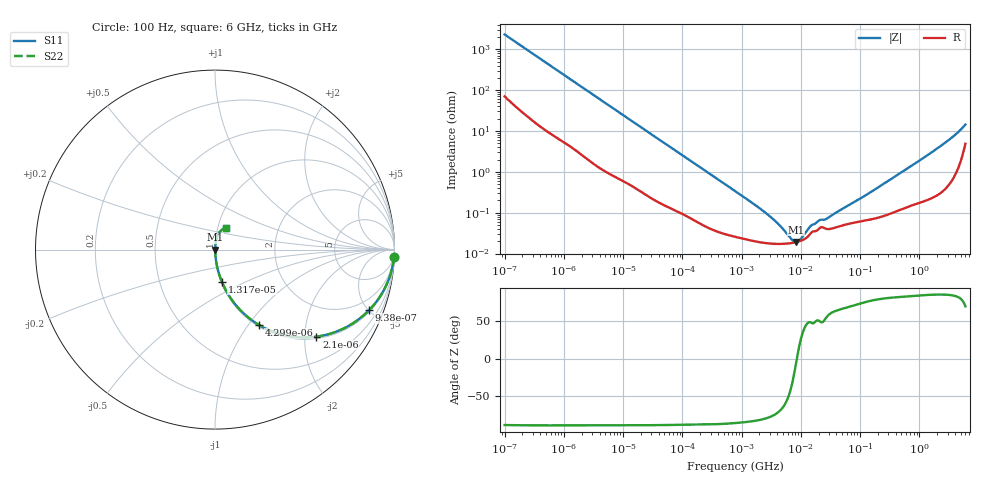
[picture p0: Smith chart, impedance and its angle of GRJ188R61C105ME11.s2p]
!Murata Part Number: GRJ188R61C105ME11
!These Parameters are Measured in Series Mode Connection
!Data Generated on Jun 19, 2026
!  o--ll--o
!Port1  Port2
!  o------o
!Operation Temp=25[degC], DC Bias Voltage=0[V]
!Freq. Start=100[Hz] Stop=6[GHz] 401[Steps]
# Hz S RI R 50
!Freq.(Hz) S11(Real) S11(Imag) S21(Real) S21(Imag) S12(Real) S12(Imag) S22(Real) S22(Imag)
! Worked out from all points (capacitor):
!   401 points, 100 Hz to 6 GHz, reference 50 ohm
!   read as one part in series: C = 687 nF near 109 Hz
!   lowest |Z| = 19 mohm at 8.312 MHz (marker M1)
!   series resonance near 8.567 MHz, so ESL is about 500 pH
!   S11 on the Smith chart (normalised r, x): 100 Hz: 2, -46; 938 Hz: 1.11, -5.05; 2.1 kHz: 1.05, -2.29; 4.299 kHz: 1.02, -1.13; 13.17 kHz: 1.01, -0.37; 6 GHz: 1.10, +0.27
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100  0.9968 -0.0432  0.00319 0.0432  0.00319 0.0432  0.9968 -0.0432
335  0.977 -0.1393  0.023 0.1393  0.023 0.1393  0.977 -0.1393
938  0.8592 -0.3369  0.1408 0.3369  0.1408 0.3369  0.8592 -0.3369
2008  0.5861 -0.4818  0.4139 0.4818  0.4139 0.4818  0.5861 -0.4818
2100  0.565 -0.4851  0.435 0.4851  0.435 0.4851  0.565 -0.4851
3005  0.3937 -0.4783  0.6063 0.4783  0.6063 0.4783  0.3937 -0.4783
4299  0.245 -0.4199  0.755 0.4199  0.755 0.4199  0.245 -0.4199
7036  0.1122 -0.3046  0.8878 0.3046  0.8878 0.3046  0.1122 -0.3046
13169  0.0379 -0.1786  0.9621 0.1786  0.9621 0.1786  0.0379 -0.1786
40335  0.00556 -0.0615  0.9944 0.0615  0.9944 0.0615  0.00556 -0.0615
774597  0.000268 -0.00338  0.9997 0.00338  0.9997 0.00338  0.000268 -0.00338
2967816  0.000176 -0.000807  0.9998 0.000807  0.9998 0.000807  0.000176 -0.000807
4440638  0.000172 -0.00045  0.9998 0.00045  0.9998 0.00045  0.000172 -0.00045
6948629  0.00018 -0.000135  0.9998 0.000135  0.9998 0.000135  0.00018 -0.000135
8311524  0.000189 -1.93e-05  0.9998 1.93e-05  0.9998 1.93e-05  0.000189 -1.93e-05
9941735  0.000204 9.68e-05  0.9998 -9.68e-05  0.9998 -9.68e-05  0.000204 9.68e-05
1.555665e7  0.000339 0.000371  0.9997 -0.000371  0.9997 -0.000371  0.000339 0.000371
2.035112e7  0.000406 0.0005  0.9996 -0.0005  0.9996 -0.0005  0.000406 0.0005
2.784235e7  0.000397 0.000605  0.9996 -0.000605  0.9996 -0.000605  0.000397 0.000605
3.124326e8  0.000962 0.00618  0.999 -0.00618  0.999 -0.00618  0.000962 0.00618
2.142435e9  0.00439 0.0396  0.9956 -0.0396  0.9956 -0.0396  0.00439 0.0396
6e9  0.0618 0.1205  0.9382 -0.1205  0.9382 -0.1205  0.0618 0.1205
